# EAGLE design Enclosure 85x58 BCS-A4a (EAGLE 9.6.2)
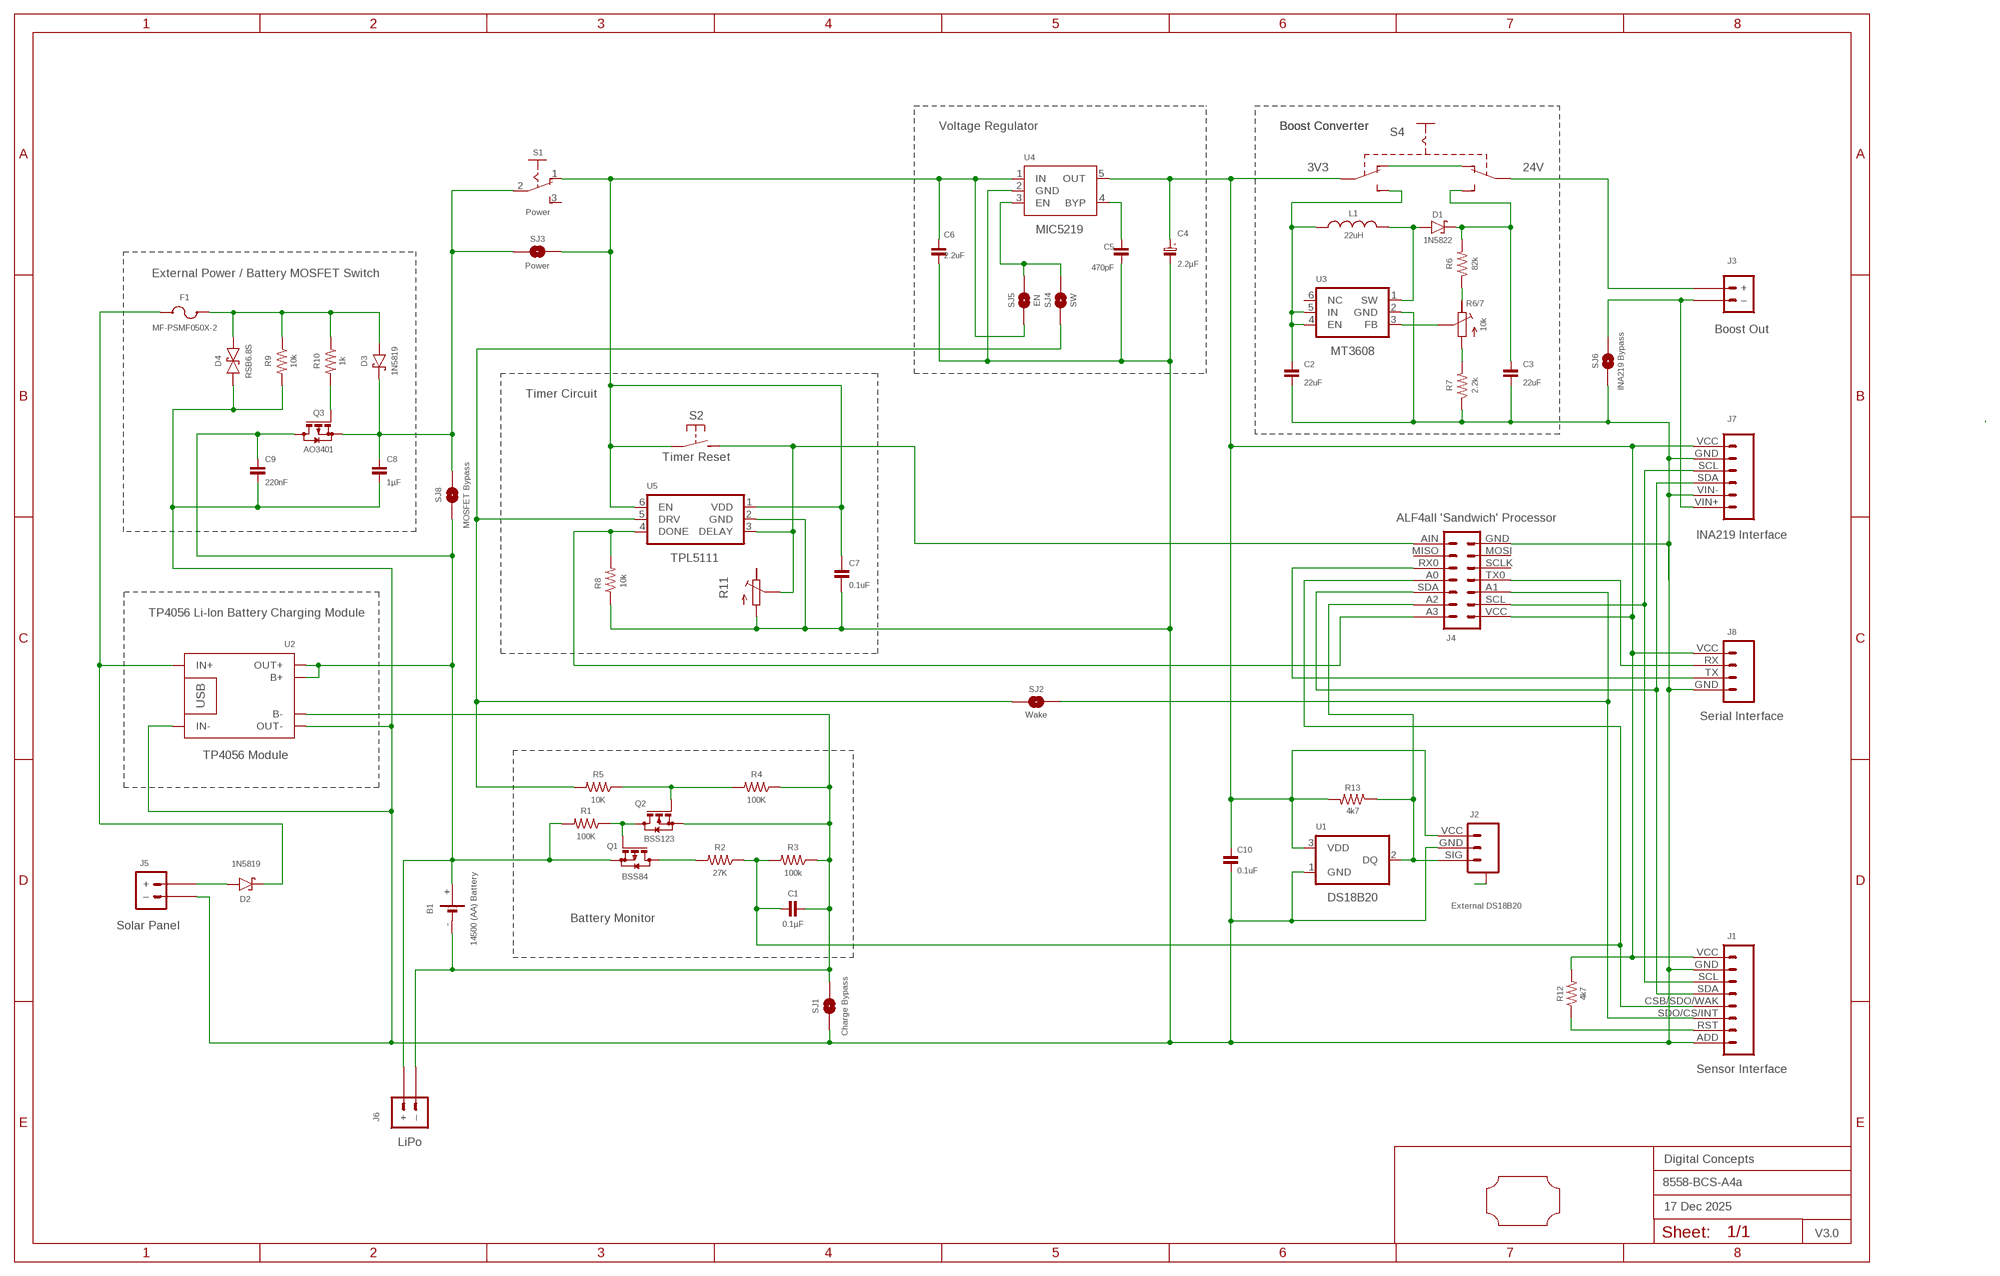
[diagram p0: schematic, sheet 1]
FRAME2 (A3L-LOC): DATE: 17 Dec 2025; OWNER: Digital Concepts; TITLE: 8558-BCS-A4a; VERSION: V3.0

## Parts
B1  14500 (AA) Battery  BATTERY-HOLDER-14500(AA)  [BATTERY-14500]
C1  0.1µF  CAPACITOR-0805  [C0805]
C2  22uF  CAPACITOR-1206  [C1206]
C3  22uF  CAPACITOR-1206  [C1206]
C4  2.2µF  CAPACITOR-1206-TANTALUM  [C1206-POLARISED]
C5  470pF  CAPACITOR-0805  [C0805]
C6  2.2uF  CAPACITOR-0805  [C0805]
C7  0.1uF  CAPACITOR  [C0805@1]
C8  1µF  CAPACITOR-0805  [C0805]
C9  220nF  CAPACITOR-0805  [C0805]
C10  0.1uF  CAPACITOR-0805  [C0805]
D1  1N5822  DIODE-SCHOTTKY-1N5822  [DIODE_SMB]
D2  1N5819  1N5819-SOD-123  [SOD-123]
D3  1N5819  DIODE-SCHOTTKY-1N5819  [SOD-123]
D4  RSB6.8S  DIODE-SCHOTTKY-BIDIRECTIONAL  [VMD2]
F1  MF-PSMF050X-2  [F0805]
J1  Sensor Interface  HEADER-1X8-SENSOR  [CONN_08-SENSOR]
J2  External DS18B20  JST-SH1.0-3-SMD-HORIZONTAL-SIG  [JST-SH1.0-3-SMD-HORIZONTAL-SIG]
J3  Boost Out  JST-GH1.25-2-HORIZONTAL-POWER  [JST-GH1.25-2-HORIZONTAL]
J4  ALF4all 'Sandwich' Processor  ALF4ALL-PROCESSOR-BOARD  [ALF4ALL-PROCESSOR-BOARD]
J5  Solar Panel  JST-PH2.0-2-VERTICAL-POWER  [JST-PH2.0-2-VERTICAL-POWER]
J6  LiPo  JST-PH2.0-2-H-POWER  [JST-PH2.0-2-HORIZONTAL-POWER]
J7  INA219 Interface  INA219-I2C-MODULE  [CONN_06-INA219]
J8  Serial Interface  HEADER-1X4-GPS  [CONN_04-GPS]
L1  22uH  INDUCTOR-CDRH104R/6D28L5038P  [CDRH104R+6D28]
Q1  BSS84  [SOT23]
Q2  BSS123  [SOT23]
Q3  AO3401  MOSFET-AO3401  [SOT-23]
R1  100K  RESISTORR0805  [R0805]
R2  27K  RESISTORR0805  [R0805]
R3  100k  RESISTORR0805  [R0805]
R4  100K  RESISTORR0805  [R0805]
R5  10K  RESISTORR0805  [R0805]
R6  82k  RESISTORR0805  [R0805]
R6/7  10k  RESISTOR-TRIMM-33  [RTRIM3*3]
R7  2.2k  RESISTOR-VIA-1  [R0805-VIA-1]
R8  10k  RESISTOR-VIA-2  [R0805-VIA-2]
R9  10k  RESISTORR0805  [R0805]
R10  1k  RESISTORR0805  [R0805]
R11  RESISTOR-TRIMM-33  [RTRIM3*3]
R12  4k7  RESISTORR0805  [R0805]
R13  4k7  RESISTORR0805  [R0805]
S1  Power  SWITCH-SLIDE-SPDT  [SWITCH-SLIDE-SPDT]
S2  Timer Reset  SWITCH-MOMENTARY-2-PIN  [SWITCH-2-PAD]
S4  SWITCH-SLIDE-DPDT-PTH-S  [SWITCH-DPDT-PTH]
SJ1  Charge Bypass  SJ-V-1  [SJ-VIA-1]
SJ2  Wake  SJ-V-1  [SJ-VIA-1]
SJ3  Power  SJ-V-1  [SJ-VIA-1]
SJ4  SW  SJ  [SJ]
SJ5  EN  SJ  [SJ]
SJ6  INA219 Bypass  SJ  [SJ]
SJ8  MOSFET Bypass  SJ  [SJ]
U1  DS18B20  [TO-92]
U2  TP4056 Module  BATTERY-CHARGER-LI-PROT  [BATTERY-CHARGER-LI-PROT]
U3  MT3608  [SOT-23-6]
U4  MIC5219  MIC5219XX  [SOT-23-5]
U5  TPL5111  TPL5111DDCR  [SOT-23-6]
U$1  PCB-OUTLINE-CA-85X58  [PROTO-28X18-OUTLINE-CA]

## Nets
A: J2.A@1(A) J2.A@3(A)
GND: C2.2 C3.2 C4.2(-) C5.2 C6.1 C7.1 C8.2 C9.2 C10.2 D4.P$2 J1.ADD J1.GND J2.GND J4.GND J5.-(–) J7.GND J7.VIN- J8.GND R7.1 R7.1@VIA R8.1 R9.2 R11.1(A) SJ1.1 SJ1.1@V SJ6.1 U1.1(GND) U2.IN- U2.OUT- U3.2(GND) U4.2(GND) U5.2(GND)
N$1: D2.A J5.+
N$2: B1.+ C9.1 J6.+ Q1.2(S) Q3.3(D) R1.2 SJ8.1 U2.B+ U2.OUT+
N$3: D2.C F1.1 U2.IN+
N$4: C8.1 D3.C Q3.2(S) S1.2(P) SJ3.2 SJ8.2
N$6: D1.A L1.2 U3.1(SW)
N$7: C5.1 U4.4(BYP)
N$8: J1.SCL J4.SCL J7.SCL
N$9: J1.RST R12.1
N$10: C1.1 J1.CSB/SDO/WAK J4.A0 R2.1 R3.2
N$11: J1.SDA J4.SDA J7.SDA
N$12: C6.2 C7.2 S1.1(O) S2.P$1(P) SJ3.1 SJ3.1@V SJ5.1 U4.1(IN) U5.1(VDD) U5.6(EN)
N$13: J2.SIG J4.A2 R13.1 U1.2(DQ)
N$14: J4.TX0 J8.RX
N$15: J3.-(–) J7.VIN+ SJ6.2
N$16: J4.RX0 J8.TX
N$19: SJ4.2 SJ5.2 U4.3(EN)
N$22: J4.A3 R8.2 R8.2@VIA U5.4(DONE)
N$23: Q1.3(D) R2.2
N$24: C2.1 L1.1 S4.P$3(S1) U3.4(EN) U3.5(IN)
N$25: J4.AIN R11.2(S) S2.P$2(S) U5.3(DELAY)
N$28: R5.2 SJ2.2 SJ4.1 U5.5(DRV)
N$30: J1.SDO/CS/INT J4.A1 SJ2.1 SJ2.1@V
N$31: C3.1 D1.C R6.2 S4.P$6(S2)
N$32: R6.1 R6/7.3(E)
N$33: R6/7.2(S) U3.3(FB)
N$34: R6/7.1(A) R7.2
N$35: Q1.1(G) Q2.3(D) R1.1
N$37: Q2.1(G) R4.2 R5.1
N$38: B1.- C1.2 J6.-(–) Q2.2(S) R3.1 R4.1 SJ1.2 U2.B-
N$39: S4.P$1(O1) S4.P$4(O2)
N$42: J3.+ S4.P$5(P2)
N$43: Q3.1(G) R10.2
N$44: D3.A D4.P$1 F1.2 R9.1 R10.1
VCC: C4.1(+) C10.1 J1.VCC J2.VCC J4.VCC J7.VCC J8.VCC R12.2 R13.2 S4.P$2(P1) U1.3(VDD) U4.5(OUT)
Unconnected: J4.MISO J4.MOSI J4.SCLK R11.3(E) S1.3(S) U3.6(NC)

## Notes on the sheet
- Voltage Regulator | Boost Converter | Boost Converter
- 3V3 | 24V
- External Power / Battery MOSFET Switch
- Timer Circuit
- TP4056 Li-Ion Battery Charging Module
- Battery Monitor

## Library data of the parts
B1 = digitalconcepts:BATTERY-HOLDER-14500(AA): 14500 (AA) battery holder
C1 C5 C6 C8-C10 = digitalconcepts:CAPACITOR-0805: 0805 Capacitor
C2 C3 = digitalconcepts:CAPACITOR-1206: 1206 Capacitor
C4 = digitalconcepts:CAPACITOR-1206-TANTALUM: Capacitor 1206 Tantalum
C7 = digitalconcepts:CAPACITOR: 0805 Capacitor
D1 = digitalconcepts:DIODE-SCHOTTKY-1N5822: 1N5822 Schottky Diode SMB
D2 = digitalconcepts:1N5819-SOD-123: 1N5819 Schottky Diode SOD-123
D3 = digitalconcepts:DIODE-SCHOTTKY-1N5819: 1N5819 Schottky Diode SOD-123
D4 = digitalconcepts:DIODE-SCHOTTKY-BIDIRECTIONAL: Schottky Bidirectional Diode
F1 = digitalconcepts:MF-PSMF050X-2: PTC Resettable Fuse
J1 = digitalconcepts:HEADER-1X8-SENSOR: IoT Sensors 1x8 Pin Header for 'Sandwich' IoT Sensors
J2 = digitalconcepts:JST-SH1.0-3-SMD-HORIZONTAL-SIG: JST SH1.0 3P SMD Horizontal Connector with Signal
J3 = digitalconcepts:JST-GH1.25-2-HORIZONTAL-POWER: JST GH1.25 2P PTH Connector (Power)
J4 = digitalconcepts:ALF4ALL-PROCESSOR-BOARD: ALF4all 'Sandwixh' Processor 2x7 Pin Header and earthed 1x1 locator pins for ALF4all 'Sandwich' Processor/RFM95W PCBs
J5 = digitalconcepts:JST-PH2.0-2-VERTICAL-POWER: JST PH2.0 2P PTH Connector (Power)
J6 = digitalconcepts:JST-PH2.0-2-H-POWER: JST PH2.0 2P Right Angle Connector with power pin labelling
J7 = digitalconcepts:INA219-I2C-MODULE: INA219 I2C Module
J8 = digitalconcepts:HEADER-1X4-GPS: NEO GPS 4-Pin Header
L1 = digitalconcepts:INDUCTOR-CDRH104R/6D28: Inductor; SPICEPREFIX: L
Q1 = digitalconcepts:BSS84: P-CHANNEL MOS FET
Q2 = digitalconcepts:BSS123: N-CHANNEL MOS FET
Q3 = digitalconcepts:MOSFET-AO3401: AO3401 P-Channel MOSFET
R1-R6 R9 R10 R12 R13 = digitalconcepts:RESISTOR: Resistor; SPICEPREFIX: R
R6/7 R11 = digitalconcepts:RESISTOR-TRIMM-3*3: Trimm Resistor - 3*3 SMD
R7 = digitalconcepts:RESISTOR-VIA-1: Resistor with via on Pad 1
R8 = digitalconcepts:RESISTOR-VIA-2: Resistor with via on Pad 2
S1 = digitalconcepts:SWITCH-SLIDE-SPDT: Mini Sliding Switch SPDT
S2 = digitalconcepts:SWITCH-MOMENTARY-2-PIN: 2 Pin Momentary Switch
S4 = digitalconcepts:SWITCH-SLIDE-DPDT-PTH-S: Switch DPDT PTH-S
SJ1-SJ3 = digitalconcepts:SJ-V-1: Solder Jumper with single Pad Via
SJ4-SJ6 SJ8 = digitalconcepts:SJ: Solder Jumper
U1 = digitalconcepts:DS18B20: Digital Thermometer -55C-125C TO92-3; AVAILABILITY: Bad; DESCRIPTION: Temperature Sensor Digital, Local -55°C ~ 125°C 12 b 8-uMAX; MF: Maxim Integrated; MP: DS18B20; PACKAGE: TO-92 Maxim Integrated; PRICE: None
U2 = digitalconcepts:BATTERY-CHARGER-LI-PROT: TP4056 Li Battery Charger module with PCB (rather than module) footprint
U3 = digitalconcepts:MT3608: MT3608 DC-DC Step-Up Voltage Converter
U4 = digitalconcepts:MIC5219XX: VOLTAGE REGULATOR; OC_FARNELL: unknown; OC_NEWARK: unknown
U5 = digitalconcepts:TPL5111DDCR: TPL5111 Nano-Power System Timer
U$1 = digitalconcepts:PCB-OUTLINE-CA-85X58: PCB outline with cut-out for 85 x 58 enclosure

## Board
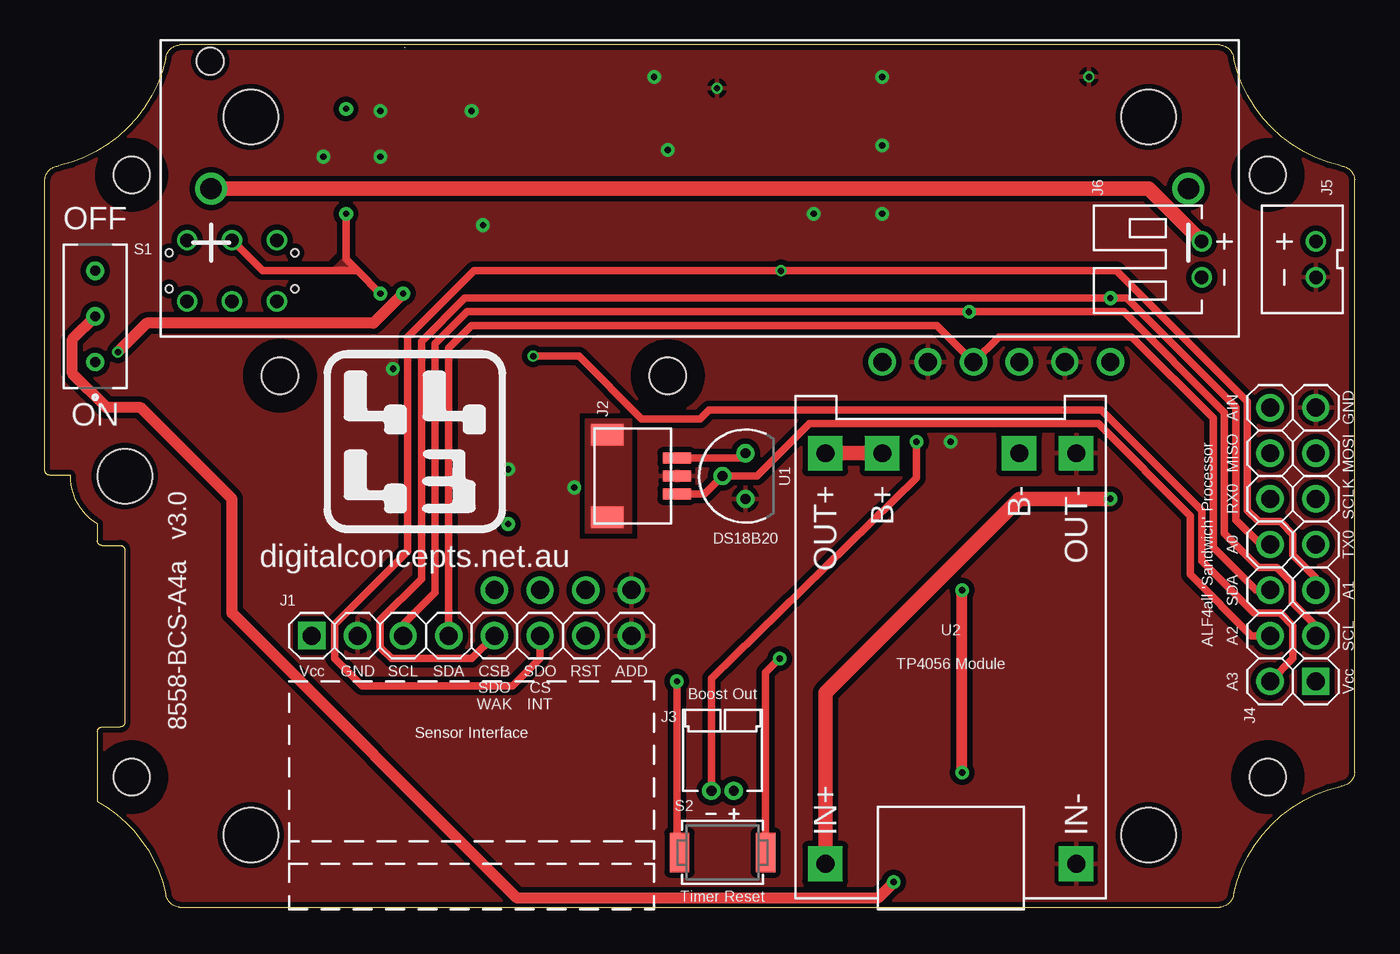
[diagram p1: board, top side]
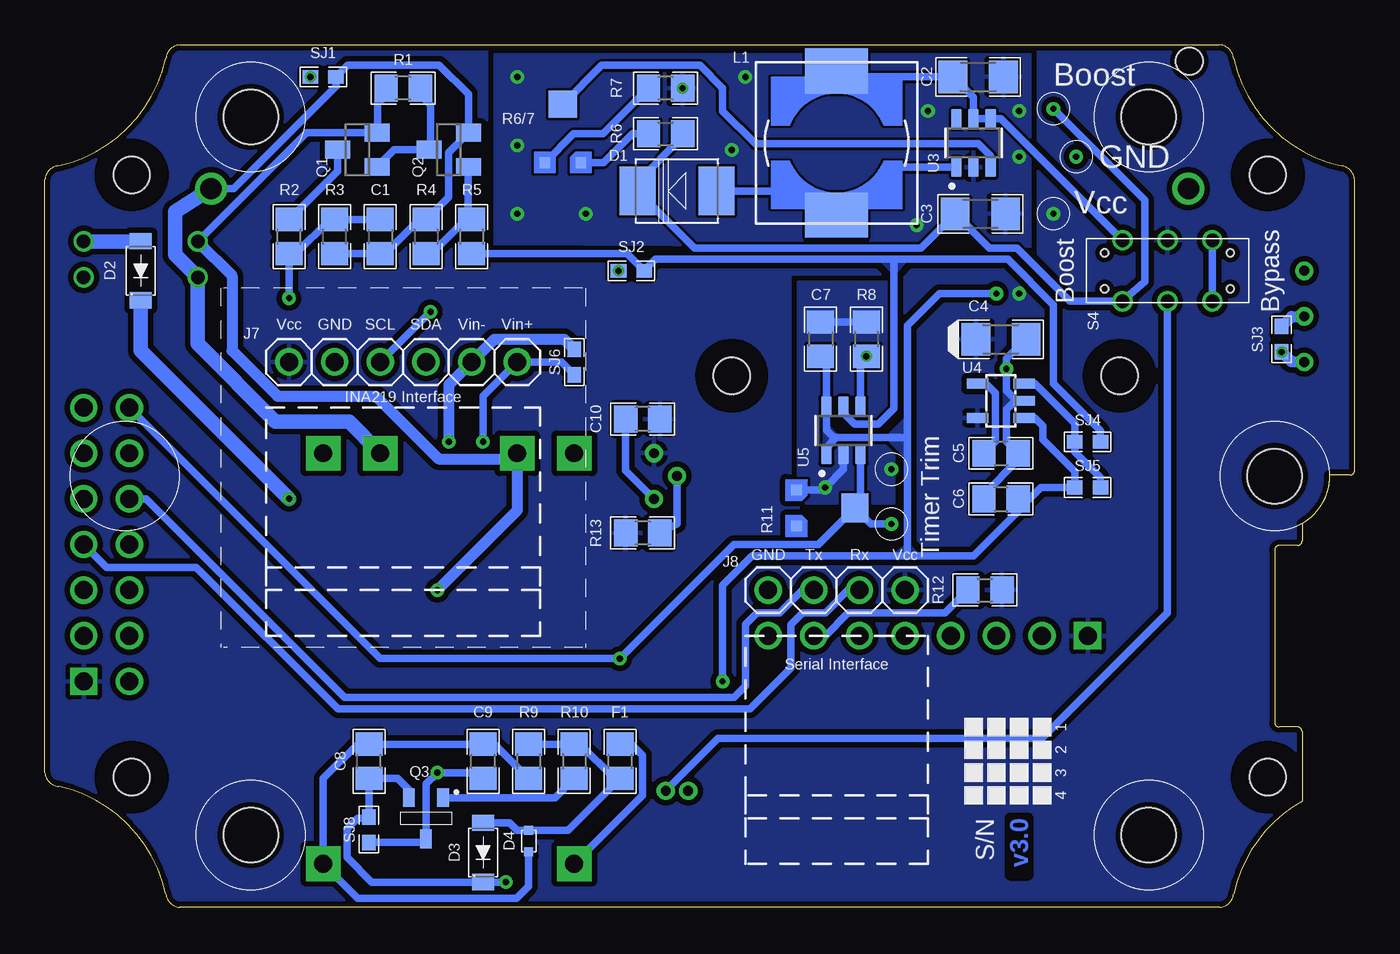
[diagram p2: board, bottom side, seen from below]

Size 72.9 x 48.01 mm. Coordinates in mm from the lower left corner, seen from the top.
Copper layers (1*16): Top 0.035mm / dielectric 1.5mm / Bottom 0.035mm
Design rules "default *": minimum track width 6mil, minimum drill 0.35mm, track to track 6mil, track to pad 6mil, pad to pad 6mil, via to via 6mil, smd to smd 6mil, copper to edge 6mil, drill to drill 6mil, minimum pad ring 1mil, minimum via ring 8mil, stop-mask expansion 4mil, vias tented up to drill 0mil, thermal gap 10mil
Holes 2.03 mm at 13.08,29.59 34.67,29.59

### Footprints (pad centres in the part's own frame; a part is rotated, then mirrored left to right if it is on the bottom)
BATTERY-14500 = drill 1.19: + -27.2,0; - 27.2,0 | hole 1.5: -27.25,7.1
C0805 = smd 1.3 x 1.5: 1 -0.95,0; 2 0.95,0
C1206 = smd 1.6 x 1.8: 1 -1.4,0; 2 1.4,0
C1206-POLARISED = smd 1.6 x 1.8: 1 -1.4,0; 2 1.4,0
C0805@1 = smd 1.3 x 1.5: 1 -0.95,0; 2 0.95,0
DIODE_SMB = smd 2 x 2.7: A 2.2,0; C -2.2,0
SOD-123 = smd 0.91 x 1.22: A -1.65,0; C 1.65,0
VMD2 = smd 0.5 x 0.5: P$1 -0.6,0; P$2 0.6,0
F0805 = smd 1.3 x 1.5: 1 -0.95,0; 2 0.95,0
CONN_08-SENSOR = drill 1 pad 1.524: ADD 17.78,0; CSB/SDO/WAK 10.16,0; GND 2.54,0; RST 15.24,0; SCL 5.08,0; SDA 7.62,0; SDO/CS/INT 12.7,0 | drill 1 pad 1.524 square: VCC 0,0
JST-SH1.0-3-SMD-HORIZONTAL-SIG = smd 1.2 x 1.8: A@1 2.3,-1.335; A@3 -2.3,-1.335 | smd 0.6 x 1.55: GND 0,2.54; SIG 1,2.54; VCC -1,2.54
JST-GH1.25-2-HORIZONTAL = drill 0.55 pad 1.016: + -0.625,0; - 0.625,0
ALF4ALL-PROCESSOR-BOARD = drill 1 pad 1.524: A0 7.62,2.54; A1 5.08,0; A2 2.54,2.54; A3 0,2.54; AIN 15.24,2.54; GND 15.24,0; MISO 12.7,2.54; MOSI 12.7,0; RX0 10.16,2.54; SCL 2.54,0; SCLK 10.16,0; SDA 5.08,2.54; TX0 7.62,0 | drill 1 pad 1.524 square: VCC 0,0
JST-PH2.0-2-VERTICAL-POWER = drill 0.75: + -1,0; - 1,0
JST-PH2.0-2-HORIZONTAL-POWER = drill 0.75: + 1,0; - -1,0
CONN_06-INA219 = drill 1 pad 1.524: GND 2.54,0; SCL 5.08,0; SDA 7.62,0; VCC 0,0; VIN+ 12.7,0; VIN- 10.16,0
CONN_04-GPS = drill 1 pad 1.524: GND 0,0; RX 5.08,0; TX 2.54,0; VCC 7.62,0
CDRH104R+6D28 = smd 2.5 x 3.5: 1 -4,0; 2 4,0
SOT23 = smd 1 x 1.4: 1 -0.95,-1.1; 2 0.95,-1.1; 3 0,1.1
SOT-23 = smd 0.65 x 1.05: 1 -0.95,-1.15; 2 0.95,-1.15; 3 0,1.15
R0805 = smd 1.3 x 1.5: 1 -0.95,0; 2 0.95,0
RTRIM3*3 = smd 0.6 x 0.6: 1 -1,-1.6; 3 1,-1.6 | smd 1.6 x 1.5: 2 0,1.65
R0805-VIA-1 = smd 1.3 x 1.5: 1 -0.95,0; 2 0.95,0 | drill 0.35 pad 0.61: 1@VIA -0.95,0
R0805-VIA-2 = smd 1.3 x 1.5: 1 -0.95,0; 2 0.95,0 | drill 0.35 pad 0.61: 2@VIA 0.95,0
SWITCH-SLIDE-SPDT = drill 0.55 pad 1.016: 1 -2.54,0; 2 0,0; 3 2.54,0
SWITCH-2-PAD = smd 1.067 x 2.184: P$1 -2.4,0; P$2 2.4,0
SWITCH-DPDT-PTH = drill 0.75: P$1 -1.7,2.5; P$2 -1.7,0; P$3 -1.7,-2.5; P$4 1.7,2.5; P$5 1.7,0; P$6 1.7,-2.5 | hole 0.42: 1,3.5; -1,3.5; 1,-3.5; -1,-3.5
SJ-VIA-1 = smd 0.864 x 0.762: 1 -0.711,0; 2 0.711,0 | drill 0.35 pad 0.61: 1@V -0.711,0
SJ = smd 0.864 x 0.762: 1 -0.711,0; 2 0.711,0
TO-92 = drill 0.55 pad 1.016: 1 -1.27,0; 2 0,1.27; 3 1.27,0
BATTERY-CHARGER-LI-PROT = drill 1 pad 1.93 square: B+ 10.795,3.81; B- 10.795,-3.81; IN+ -12.065,6.985; IN- -12.065,-6.985; OUT+ 10.795,6.985; OUT- 10.795,-6.985
SOT-23-6 = smd 1.1 x 0.6: 1 -1.35,0.95; 2 -1.35,0; 3 -1.35,-0.95; 4 1.35,-0.95; 5 1.35,0; 6 1.35,0.95
SOT-23-5 = smd 0.55 x 1.2: 1 -0.95,-1.3; 2 0,-1.3; 3 0.95,-1.3; 4 0.95,1.3; 5 -0.95,1.3
PROTO-28X18-OUTLINE-CA = hole 2.032: -31.623,16.764; -31.623,-16.764; 31.623,-16.764; 31.623,16.764 | hole 3.048: -24.994,19.99; -32.004,0; -24.994,-19.99; 24.994,-19.99; 24.994,19.99

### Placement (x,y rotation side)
B1  36.45,40.01 0 top
C1  54.23,37.34 270 bottom
C2  20.95,46.23 0 bottom
C3  20.83,38.61 0 bottom
C4  19.68,31.62 0 bottom
C5  19.68,25.27 0 bottom
C6  19.68,22.73 0 bottom
C7  29.72,31.62 270 bottom
C8  54.86,8.13 90 bottom
C9  48.51,8.13 90 bottom
C10  39.62,27.18 180 bottom
D1  37.72,39.88 0 bottom
D2  67.56,35.43 270 bottom
D3  48.51,3.05 270 bottom
D4  45.97,3.68 270 bottom
F1  40.89,8.13 270 bottom
J1  14.86,15.11 0 top
J2  32.64,24 270 top
J3  37.72,6.48 180 top
J4  70.74,12.57 90 top
J5  70.74,36.07 270 top
J6  64.39,36.07 90 top
J7  59.31,30.35 0 bottom
J8  32.64,17.65 0 bottom
L1  28.83,42.55 270 bottom
Q1  55.5,42.16 90 bottom
Q2  50.42,42.16 90 bottom
Q3  51.69,4.95 180 bottom
R1  52.96,45.59 180 bottom
R2  59.31,37.34 90 bottom
R3  56.77,37.34 90 bottom
R4  51.69,37.34 270 bottom
R5  49.15,37.34 270 bottom
R6  38.35,43.05 0 bottom
R6/7  44.07,43.05 0 bottom
R7  38.35,45.59 180 bottom
R8  27.18,31.62 270 bottom
R9  45.97,8.13 270 bottom
R10  43.43,8.13 270 bottom
R11  29.46,22.23 270 bottom
R12  20.57,17.65 0 bottom
R13  39.62,20.83 180 bottom
S1  2.79,32.89 90 top
S2  37.72,3.05 0 top
S4  10.41,35.43 270 bottom
SJ1  57.4,46.23 0 bottom
SJ2  40.26,35.43 0 bottom
SJ3  4.06,31.62 90 bottom
SJ4  14.86,25.91 180 bottom
SJ5  14.86,23.37 0 bottom
SJ6  43.43,30.35 270 bottom
SJ8  54.86,4.32 90 bottom
U1  38.99,24 90 top
U2  50.42,14.48 90 top
U3  21.21,42.55 90 bottom
U4  19.68,28.19 90 bottom
U5  28.45,26.54 90 bottom
U$1  36.45,24 0 top

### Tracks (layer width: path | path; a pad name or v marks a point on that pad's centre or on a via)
$X1
  cutout Bottom: 68.07,42.8 arc180 68.07,38.73 arc180
$X2
  cutout Bottom: 68.07,9.27 arc180 68.07,5.21 arc180
$X3
  cutout Bottom: 4.83,9.27 arc180 4.83,5.21 arc180
$X4
  cutout Top: 4.83,42.8 arc180 4.83,38.73 arc180
$X5
  cutout Bottom: 4.83,42.8 arc180 4.83,38.73 arc180
$X6
  cutout Top: 68.07,42.8 arc180 68.07,38.73 arc180
$X7
  cutout Top: 68.07,9.27 arc180 68.07,5.21 arc180
$X8
  cutout Top: 4.83,9.27 arc180 4.83,5.21 arc180
$X9
  cutout Bottom: 13.08,31.62 arc180 13.08,27.56 arc180
$X10
  cutout Top: 13.08,31.62 arc180 13.08,27.56 arc180
A
  pour Top (no thermals): 30.1,27.18 32.64,27.18 32.64,20.83 30.1,20.83
GND  (via drill 0.35)
  Bottom 0.406: R8.1 C7.1 | C4.2 19.38,30.53 v19.38,29.97 19.38,28.76 18.81,28.19 U4.2 18.89,28.19 19.38,27.71 19.38,25.91 C5.2 18.73,24.89 20.63,22.99 C6.1 | C10.2 40.57,24.32 U1.1 | R11.1 29.61,23.23 v29.46,23.37 28.45,24.38 U5.2 | R9.2 46.87,8.07 47.88,9.08 C9.2 C8.2 55.5,9.08 57.4,7.18 U2.IN- 55.5,0.51 46.64,0.51 45.97,1.18 D4.P$2
  Bottom 0.61: SJ6.1 43.99,31.62 47.88,31.62 J7.VIN- 50.42,29.08 v50.42,25.91
  other vias: 46.61,38.61 18.67,41.78 33.91,46.23 24.38,37.97 46.61,46.23 15.49,41.78 18.67,44.32 23.75,44.32 34.67,42.16 42.8,38.61 46.61,42.42 25.78,24.38
  pour Top (isolate 0.305, rank 5): -2.08,49.93 -2.08,-1.97 74.92,-1.97 74.92,49.93
  pour Bottom: 47.88,47.5 47.88,36.92 18.03,36.75 18.03,47.5
  pour Bottom (no thermals): 19.38,28.76 18.81,28.19 19.38,27.71
  pour Bottom (rank 2, no thermals): 30.99,34.8 25.65,34.8 25.65,22.48 30.99,22.48
N$1
  Bottom 0.813: D2.A 67.58,37.07 J5.+
N$2  (via drill 0.35)
  Top 0.61: v51.05,7.49 v51.05,17.65
  Top 0.813: U2.B+ U2.OUT+ | J6.+ 61.45,40.01 B1.+
  Bottom 0.406: R1.2 53.91,45.19 54.37,44.73 54.37,43.15 Q1.2 58.34,43.11 J6.+ | SJ8.1 51.88,3.61 Q3.3 51.69,6.86 v51.05,7.49 48.83,7.49 C9.1
  Bottom 0.61: v51.05,17.65 46.61,22.1 U2.B+ 46.93,24.96 50.99,24.96 54.48,28.45 59.94,28.45 62.48,30.99 62.48,35.16 J6.+
N$3  (via drill 0.35)
  Top 0.813: U2.IN+ 43.43,11.94 54.23,22.73 v59.31,22.73
  Bottom 0.406: U2.IN+ 39.62,6.22 39.62,8.44 40.26,9.08 F1.1
  Bottom 0.813: D2.C 67.56,30.99 v59.31,22.73
N$4  (via drill 0.35)
  Top 0.61: v47.24,1.4 46.35,0.51 26.29,0.51 10.41,16.38 10.41,22.73 5.33,27.81 3.43,27.81 1.52,29.72 1.52,31.62 S1.2
  Bottom 0.406: Q3.2 52.64,6.54 53.28,7.18 C8.1 SJ8.2 54.94,4.95 55.5,4.95 56.08,4.37 56.08,2.77 54.71,1.4 D3.C v47.24,1.4
  Bottom 0.61: SJ3.2 3.5,32.89 S1.2
N$6
  Bottom 0.406: D1.A 30.8,39.88 29.46,38.55 L1.2 28.19,38.55 25.54,41.2 U3.1
N$7
  Bottom 0.406: C5.1 19.99,25.91 19.99,28.63 20.45,29.08 20.92,29.08 U4.4
N$8  (via drill 0.35)
  Top 0.406: J4.SCL 70.74,15.67 69.44,16.97 69.44,18.06 68.58,18.92 67.54,18.92 65.66,20.8 65.66,27.53 60.05,33.15 v51.44,33.15 23.49,33.15 21.72,31.37 21.72,17.53 19.94,15.75 J1.SCL
  Bottom 0.406: v51.44,33.15 J7.SCL
N$9
  Bottom 0.406: J1.RST 29.46,15.11 28.19,16.38 22.79,16.38 R12.1
N$10  (via drill 0.35)
  Top 0.406: J1.CSB/SDO/WAK 23.75,13.84 19.3,13.84 18.67,14.48 18.67,16 20.95,18.29 20.95,31.5 23.37,33.91 v59.31,33.91 60.22,33.91 66.29,27.84 66.29,21.57 67.67,20.19 J4.A0
  Bottom 0.406: v59.31,33.91 R2.1 58.93,36.39 57.03,38.29 R3.2 C1.1
N$11
  Top 0.406: J4.SDA 67.41,17.65 65.02,20.04 65.02,27.23 60.5,31.75 53.09,31.75 J7.SDA 49.66,32.39 23.75,32.39 22.48,31.12 J1.SDA
N$12  (via drill 0.35)
  Top 0.406: v35.18,12.57 35.18,3.44 S2.P$1
  Top 0.61: v19.94,34.16 18.29,32.51 5.66,32.51 SJ3.1@V
  Bottom 0.406: C7.2 29.4,30.1 U5.6 29.4,26.57 28.91,26.09 | 24.89,26.16 28.83,26.16 28.91,26.09 | v19.94,34.16 23.11,34.16 24.89,32.39 24.89,26.16 | U4.1 17.79,27.24 17.35,26.8 17.35,26.04 15.57,24.26 SJ5.1 17.47,23.37 18.11,22.73 C6.2 18.73,22.03 21.21,19.56 24.89,19.56 | U5.1 29.4,25.6 28.91,26.09 | 24.89,19.56 33.53,19.56 35.18,17.91 v35.18,12.57 | 24.89,19.56 24.89,26.16
  Bottom 0.61: SJ3.1@V 3.5,30.35 S1.1
  pour Bottom (no thermals): 29.4,26.7 28.84,26.14 29.4,25.57
  pour Bottom (no thermals): 25.9,26.15 24.89,25.15 24.89,27.15
  pour Bottom (no thermals): 24.89,20.07 24.38,19.56 25.53,19.56
N$13
  Top 0.406: J4.A2 67.16,15.11 63.75,18.52 63.75,21.79 58.62,26.92 42.54,26.92 39.62,24 U1.2 36.72,23 J2.SIG
  Bottom 0.406: U1.2 37.72,21.34 R13.1
N$14
  Bottom 0.406: J8.RX 28.19,17.65 29.46,16.38 30.73,16.38 31.37,15.75 31.37,13.34 33.65,11.05 56.57,11.05 64.48,18.92 69.47,18.92 J4.TX0
N$15  (via drill 0.35)
  Top 0.406: J3.- 37.09,12.73 48.51,23.89 v48.51,25.91
  Bottom 0.406: SJ6.2 44.14,30.35 J7.VIN+ 48.51,28.45 v48.51,25.91
N$16
  Bottom 0.406: J4.RX0 67.26,22.73 56.21,11.68 34.54,11.68 33.91,12.32 33.91,15.75 33.27,16.38 32,16.38 30.73,17.65 J8.TX
N$19
  Bottom 0.406: U4.3 17.79,29.14 15.57,26.92 SJ4.2 15.57,25.35 14.15,23.93 SJ5.2
N$22
  Top 0.406: R8.2@VIA 29.72,30.67 33.21,27.18 36.45,27.18 36.96,27.69 58.8,27.69 64.39,22.1 64.39,19.28 67.28,16.38 68.76,16.38 69.47,15.67 69.47,13.84 J4.A3
  Bottom 0.406: R8.2@VIA 27.5,30.1 U5.4
N$23
  Bottom 0.406: Q1.3 56.62,41.77 56.62,40.98 R2.2
N$24
  Bottom 0.406: L1.1 28.51,46.23 C2.1 | C2.1 | C2.1 21.21,45.08 U3.5 U3.4 19.68,43.9 S4.P$3
N$25  (via drill 0.35)
  Top 0.406: v40.89,13.84 40.12,13.07 S2.P$2
  Bottom 0.406: J4.AIN 54.23,13.84 v40.89,13.84 34.54,20.19 29.85,20.19 R11.2 | U5.3 27.5,22.54 R11.2 | R11.2 26.92,21.34 v25.78,21.34
N$28
  Bottom 0.406: U5.5 28.45,27.51 27.84,26.9 26.5,26.9 25.65,27.75 25.65,36.07 | R5.2 40.5,36.39 SJ2.2 38.91,36.07 25.65,36.07 | SJ4.1 14.15,26.54 16.76,29.16 16.76,33.53 19.3,36.07 25.65,36.07
  pour Bottom (no thermals): 25.02,36.07 26.29,36.07 25.65,35.43
N$30
  Top 0.406: J4.A1 70.74,18.34 69.47,19.61 69.47,20.75 68.76,21.46 67.56,21.46 66.93,22.1 66.93,28.14 59.64,35.43 SJ2.1@V 23.88,35.43 20.19,31.75 20.19,19.81 16.13,15.75 16.13,13.84 17.65,12.32 26.03,12.32 27.56,13.84 J1.SDO/CS/INT
N$31  (via drill 0.35)
  Bottom 0.406: R6.2 37.4,42.89 39.92,40.38 D1.C 36.74,36.7 24.13,36.7 C3.1 20.32,36.7 18.8,36.7 15.83,33.73 S4.P$6 11.68,34.83 11.68,39.37 v16.76,44.45
N$32
  Bottom 0.406: R6/7.3 41.8,41.45 40.2,43.05 R6.1
N$33
  Bottom 0.406: R6/7.2 41.91,46.86 36.45,46.86 35.18,45.59 35.18,44.32 33.36,42.5 20.93,42.5 20.26,41.83 U3.3
N$34
  Bottom 0.406: R7.2 41.84,43.05 43.47,43.05 R6/7.1
N$35
  Bottom 0.406: R1.1 52.01,45.21 51.44,44.65 51.44,42.24 Q2.3 53.45,42.16 Q1.1
N$37
  Bottom 0.406: R4.2 51.37,36.39 49.47,38.29 R5.1 49.35,38.49 49.35,41.18 Q2.1
N$38
  Bottom 0.406: B1.- 62.38,40.01 56.69,45.7 SJ1.2 56.06,46.86 50.95,46.86 49.32,45.25 Q2.2 50.43,42 50.43,39.54 R4.1 52.07,38.29 53.97,36.39 C1.2 R3.1
  Bottom 0.813: U2.B- 55.97,27.05 60.07,27.05 64.39,31.37 J6.- 65.66,36.34 65.66,38.73 B1.-
N$39
  Bottom 0.406: S4.P$1 S4.P$4
N$42
  Bottom 0.406: J3.+ 35.42,9.4 17.4,9.4 10.41,16.38 S4.P$5
N$43
  Bottom 0.406: Q3.1 44.51,6.1 R10.2
N$44
  Bottom 0.406: D3.A 47.02,4.7 46.61,4.28 D4.P$1 43.79,4.28 F1.2 41.2,7.18 43.1,9.08 R10.1 R9.1
VCC  (via drill 0.35)
  Top 0.406: v16.76,38.61 16.76,36.07 17.4,35.43 | v18.67,34.16 17.4,35.43 | 17.4,35.43 12.11,35.43 S4.P$2 | U1.3 38.72,25 J2.VCC
  pour Bottom (isolate 0.305, rank 5): -1.08,48.93 -1.08,-0.97 73.92,-0.97 73.92,48.93
  pour Top (rank 2, no thermals): 16.76,35.43 16.76,36.07 16.13,35.43
X$1
  cutout Bottom: 13.08,31.62 arc-180 13.08,27.56 arc-180
X$2
  cutout Top: 13.08,31.62 arc-180 13.08,27.56 arc-180
X$3
  cutout Top: 34.67,31.62 arc-180 34.67,27.56 arc-180
X$4
  cutout Bottom: 34.67,31.62 arc-180 34.67,27.56 arc-180

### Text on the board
Bottom: v3.0
tPlace: OFF | ON | AIN | GND | MISO | MOSI | RX0 | SCLK | A0 | TX0 | digitalconcepts.net.au | SDA | A1 | 8558-BCS-A4a v3.0 | A2 | SCL | Vcc | GND | SCL | SDA | RST | ADD | A3 | Vcc | CSB / SDO / WAK | SDO / CS / INT
bPlace: Boost | GND | Vcc | Vin+ | Vin- | SDA | SCL | GND | Vcc | Timer Trim | Vcc | Rx | Tx | GND | 1 | 2 | 3 | 4 | S/N
tNames: TP4056 Module
bNames: Bypass | Boost
bValues: Charge / Bypass | Bypass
